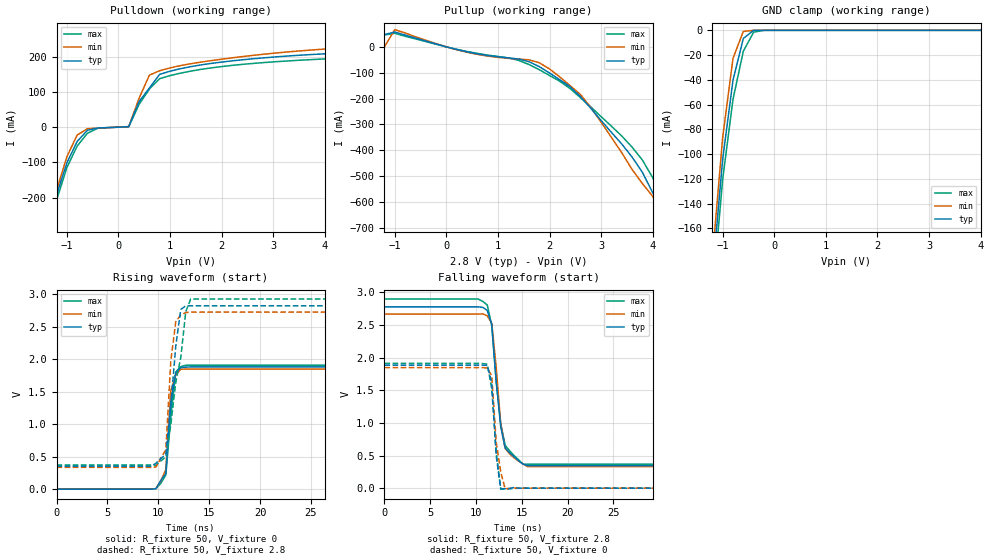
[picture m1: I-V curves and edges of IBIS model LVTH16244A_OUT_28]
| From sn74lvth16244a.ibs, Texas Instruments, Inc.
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|  Model  LVTH16244A OUTPUT_28
[Model]   LVTH16244A_OUT_28
Model_type  3-state
Polarity   Inverting
Enable   Active-Low
Vmeas = 1.5V
Cref = 50pF
Rref = 500
Vref = 0
| variable   typ   min   max
C_comp   9pf   NA   NA
[Temperature Range]   40   -25   100
| Ambient temperature   25   -40   85
[Voltage range]   2.8   2.7   2.9
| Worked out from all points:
|   slope of the pulldown table from 0 to 0.42 V, typ, clamps not added: 5.5 ohm
|   slope of the pullup table from 0 to 0.42 V, typ, clamps not added: 21.2 ohm
|   GND clamp passes 1 mA (typ) near -0.43 V on its own axis
|   rising waveform, R_fixture 50, V_fixture 0: 20-80 % time 606ps typ, 447ps min, 692ps max; typ from 0.004 V to 1.88 V
|   falling waveform, R_fixture 50, V_fixture 2.8: 20-80 % time 1.02ns typ, 979ps min, 1.09ns max; typ from 2.78 V to 0.35 V
|   rising waveform, R_fixture 50, V_fixture 2.8: 20-80 % time 885ps typ, 636ps min, 1.36ns max; typ from 0.357 V to 2.82 V
|   falling waveform, R_fixture 50, V_fixture 0: 20-80 % time 560ps typ, 732ps min, 646ps max; typ from 1.89 V to 0.004 V
[Pullup]
|   Voltage   I(typ)   I(min)   I(max)
-5V       62.11uA    60.61uA    61.62uA
-2V       53.06uA    50.33uA    53.74uA
-1.8V     52.82uA    50.14uA    42.27mA
-1.4V     52.37uA    49.71uA    44.2mA
-1.2V     47.72mA    49.51uA    46.1mA
-1V       57.53mA    66.51mA    52.62mA
1.8V      -76.31mA   -61.37mA   -88.15mA
2.6V      -193.1mA   -184.3mA   -196.5mA
3.6V      -426.3mA   -474.3mA   -388mA
4.4V      -701.7mA   -750.1mA   -661.3mA
4.6V      -781.1mA   -841.9mA   -728.2mA
10V       -2.925A    -3.321A    -2.54A
[Pulldown]
|   Voltage   I(typ)   I(min)   I(max)
-5V       -2.914A    -3.263A    -2.657A
-1.4V     -304.8mA   -304mA     -319.2mA
-1V       -101.5mA   -84.01mA   -114.9mA
-800mV    -40.6mA    -22.5mA    -53.57mA
-400mV    -2.476mA   -2.814mA   -3.202mA
200mV     1.401mA    1.629mA    1.235mA
400mV     72.36mA    81.83mA    64.42mA
600mV     110.8mA    147.3mA    108mA
1V        158.5mA    167.9mA    146.1mA
2.8V      196.1mA    206.3mA    182.7mA
7.6V      250.1mA    284.1mA    221.2mA
10V       307.2mA    341.3mA    254.8mA
[GND Clamp]
|   Voltage   I(typ)   I(min)   I(max)
-5V       -2.882A    -3.187A    -2.626A
-1.2V     -198.7mA   -184.3mA   -215mA
-1V       -104.1mA   -86.44mA   -120.3mA
-800mV    -40.32mA   -22.61mA   -55.75mA
-600mV    -6.507mA   -890.7uA   -16.88mA
-400mV    -72.46uA   -1.131uA   -1.492mA
-200mV    -80.35nA   -571.5pA   -9.081uA
5V        19.66nA    201.4pA    99.5nA
[ramp]
| variable   typ   min   max
dV/dt_r   1.158E-00/7.150E-10  1.152E-00/3.920E-10  1.206E-00/7.650E-10
dV/dt_f   1.476E+00/5.080E-10  1.410E+00/4.430E-10  1.530E+00/6.140E-10
R_load = 50
[Rising Waveform]
R_fixture = 50
V_fixture = 0
V_fixture_min = 0
V_fixture_max = 0
C_fixture = 0
L_fixture = 0
|   Time   V(typ)   V(min)   V(max)
0s        4.006mV    4.066mV    3.915mV
9.277ns   4.006mV    4.066mV    3.915mV
9.766ns   10.07mV    12.89mV    10.85mV
10.25ns   138.9mV    131.9mV    93.08mV
10.74ns   244.7mV    304.9mV    219.4mV
11.23ns   1.345V     1.518V     1.118V
11.72ns   1.798V     1.762V     1.807V
12.21ns   1.873V     1.848V     1.888V
12.7ns    1.88V      1.85V      1.91V
49.71ns   1.884V     1.85V      1.91V
[Falling Waveform]
R_fixture = 50
V_fixture = 2.8
V_fixture_min = 2.7
V_fixture_max = 2.9
C_fixture = 0pf
L_fixture = 0nH
|   Time   V(typ)   V(min)   V(max)
0s        2.777V     2.667V     2.896V
10.25ns   2.777V     2.667V     2.896V
11.23ns   2.722V     2.64V      2.805V
11.72ns   2.509V     2.527V     2.489V
12.21ns   1.638V     1.85V      1.628V
12.7ns    943mV      982.2mV    993.1mV
13.18ns   620.4mV    613.7mV    661.5mV
15.14ns   372.5mV    374.6mV    370.2mV
15.63ns   350.1mV    335.1mV    370.8mV
49.71ns   350.1mV    335.1mV    370.8mV
[Rising Waveform]
R_fixture = 50
V_fixture = 2.8
V_fixture_min = 2.7
V_fixture_max = 2.9
C_fixture = 0pf
L_fixture = 0nH
|   Time   V(typ)   V(min)   V(max)
0s        357mV      339.9mV    375.5mV
9.277ns   357mV      338.8mV    375.5mV
9.766ns   401.4mV    344.5mV    370.4mV
10.74ns   537.6mV    608.4mV    500.8mV
11.23ns   1.297V     1.977V     998.1mV
11.72ns   2.208V     2.581V     1.65V
12.21ns   2.768V     2.685V     2.03V
12.7ns    2.823V     2.719V     2.733V
13.18ns   2.823V     2.726V     2.927V
49.71ns   2.823V     2.726V     2.927V
[Falling Waveform]
R_fixture = 50
V_fixture = 0
V_fixture_min = 0
V_fixture_max = 0
C_fixture = 0pf
L_fixture = 0nH
|   Time   V(typ)   V(min)   V(max)
0s        1.885V     1.848V     1.912V
10.25ns   1.885V     1.848V     1.912V
11.23ns   1.882V     1.842V     1.901V
11.72ns   1.606V     1.724V     1.521V
12.21ns   495.5mV    707.1mV    550.5mV
12.7ns    -3.658mV   252.8mV    -10.57mV
13.18ns   -3.842mV   -4.28mV    -10.1mV
14.16ns   16.68mV    7.904mV    -557uV
14.65ns   4.073mV    4.168mV    3.957mV
49.71ns   4.073mV    4.167mV    3.957mV
